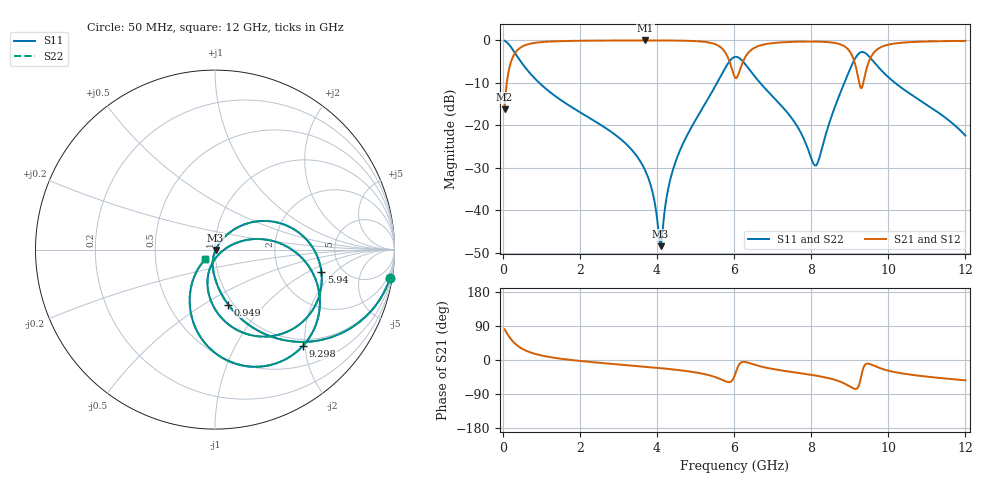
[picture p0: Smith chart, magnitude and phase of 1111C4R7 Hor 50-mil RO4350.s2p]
# GHz S MA R 50
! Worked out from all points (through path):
!   11951 points, 50 MHz to 12 GHz, reference 50 ohm
!   highest |S21| = -0.03 dB at 3.703 GHz (marker M1); lowest = -16.3 dB at 50 MHz (marker M2)
!   group delay of S21, straight-line fit = 15.9 ps
!   lowest |S11| = -48.5 dB at 4.093 GHz (marker M3), VSWR 1.01, Z = 50.3 - j0.154 ohm
!   |S11| at or under -10 dB: 946.8 MHz to 5.56 GHz (4.614 GHz wide, 142 % of centre); 6.675 GHz to 8.861 GHz (2.186 GHz wide, 28.1 % of centre); 10.17 GHz to end of sweep
!   |S22| runs from -48.5 to -0.1 dB; largest |S21 - S12| = 0
!   S11 on the Smith chart (normalised r, x): 50 MHz: 1, -12; 949 MHz: 0.95, -0.64; 5.94 GHz: 3.48, -1.39; 9.298 GHz: 0.86, -1.95; 12 GHz: 0.89, -0.10
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0.05  0.9881 -9.1  0.1536 80.9  0.1536 80.9  0.9881 -9.1
0.304  0.726 -45.0  0.6872 44.9  0.6872 44.9  0.726 -45.0
0.949  0.3155 -76.5  0.9479 13.3  0.9479 13.3  0.3155 -76.5
2.042  0.1391 -92.3  0.9887 -2.9  0.9887 -2.9  0.1391 -92.3
3.703  0.0289 -102.4  0.9966 -17.9  0.9966 -17.9  0.0289 -102.4
4.034  0.006048 -74.8  0.9962 -20.9  0.9962 -20.9  0.006048 -74.8
4.093  0.003774 -24.0  0.996 -21.5  0.996 -21.5  0.003774 -24.0
4.307  0.01922 52.1  0.9949 -23.7  0.9949 -23.7  0.01922 52.1
4.553  0.04515 55.3  0.9923 -26.4  0.9923 -26.4  0.04515 55.3
5.617  0.3524 26.5  0.852 -49.2  0.852 -49.2  0.3524 26.5
5.94  0.6064 -12.0  0.4679 -55.4  0.4679 -55.4  0.6064 -12.0
6.025  0.6383 -26.8  0.3665 -38.8  0.3665 -38.8  0.6383 -26.8
6.232  0.5634 -59.3  0.5604 -4.9  0.5604 -4.9  0.5634 -59.3
6.615  0.3404 -89.1  0.8514 -14.9  0.8514 -14.9  0.3404 -89.1
7.565  0.1095 -105.2  0.9615 -32.6  0.9615 -32.6  0.1095 -105.2
8.017  0.03926 -74.0  0.967 -39.4  0.967 -39.4  0.03926 -74.0
8.177  0.03691 -22.1  0.9648 -42.2  0.9648 -42.2  0.03691 -22.1
8.912  0.3602 5.8  0.8196 -64.6  0.8196 -64.6  0.3602 5.8
9.298  0.7266 -47.7  0.2735 -43.3  0.2735 -43.3  0.7266 -47.7
9.608  0.5694 -90.8  0.6994 -14.2  0.6994 -14.2  0.5694 -90.8
10.009  0.3658 -112.0  0.8908 -28.3  0.8908 -28.3  0.3658 -112.0
12  0.07548 -134.5  0.9846 -53.7  0.9846 -53.7  0.07548 -134.5
